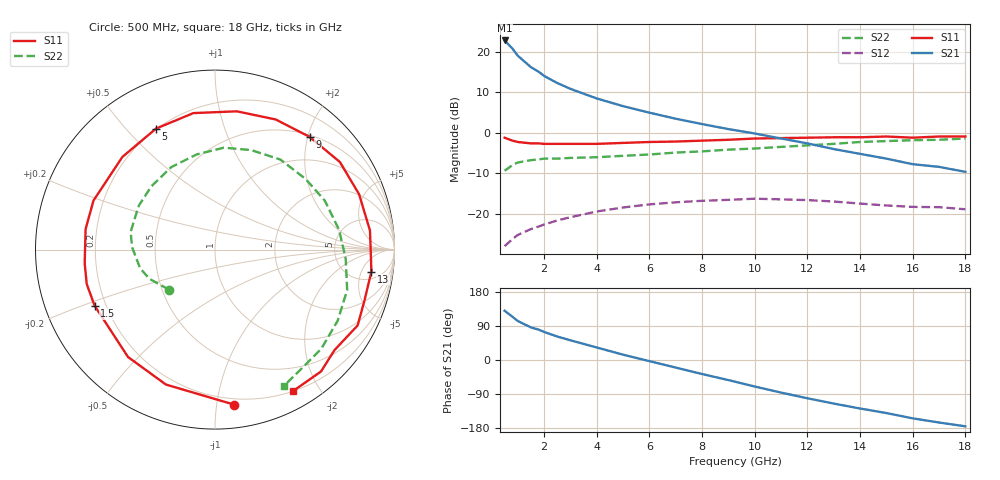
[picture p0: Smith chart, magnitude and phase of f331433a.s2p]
!ATF-33143
!S-PARAMETERS at Vds=3V  Id=60mA.  LAST UPDATED 09-29-99
# ghz s ma r 50
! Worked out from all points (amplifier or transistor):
!   23 points, 500 MHz to 18 GHz, reference 50 ohm
!   highest |S21| = 22.8 dB at 500 MHz (marker M1)
!   |S21| within 3 dB of that: start of sweep to 912.4 MHz
!   unconditionally stable (mu >= 1): 3.853 GHz to end of sweep
!   at 1.5 GHz: K = 0.66, MSG = 20.0 dB, |S12| = -23.7 dB
!   at 7 GHz: K = 1.12, MAG = 8.2 dB, |S12| = -17.1 dB
!   at 18 GHz: K = 1.44, MAG = 0.7 dB, |S12| = -18.9 dB
!   lowest NFmin = 0.11 dB at 500 MHz
!   S11 on the Smith chart (normalised r, x): 500 MHz: 0.16, -1.12; 1.5 GHz: 0.16, -0.22; 5 GHz: 0.20, +0.61; 9 GHz: 0.53, +2.03; 13 GHz: 7, -8; 18 GHz: 0.20, -1.68
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0.5  0.87 -83.0  13.75 130.0  0.04 52.0  0.34 -139.0
0.8  0.8 -110.0  10.89 114.0  0.049 43.0  0.4 -156.0
1  0.77 -129.0  8.92 103.0  0.055 38.0  0.43 -166.0
1.5  0.74 -155.0  6.44 86.0  0.065 32.0  0.46 179.0
1.8  0.74 -165.0  5.64 80.0  0.07 30.0  0.47 173.0
2  0.73 -174.0  5.02 74.0  0.074 29.0  0.48 168.0
2.5  0.73 171.0  4.11 62.0  0.083 25.0  0.48 158.0
3  0.73 158.0  3.48 52.0  0.091 20.0  0.49 150.0
4  0.73 135.0  2.65 33.0  0.107 11.0  0.5 135.0
5  0.75 116.0  2.13 14.0  0.12 0.0  0.52 118.0
6  0.77 99.0  1.77 -3.0  0.131 -12.0  0.54 101.0
7  0.78 81.0  1.49 -20.0  0.139 -25.0  0.57 85.0
8  0.8 65.0  1.28 -37.0  0.145 -37.0  0.59 70.0
9  0.82 50.0  1.11 -53.0  0.149 -50.0  0.62 54.0
10  0.85 35.0  0.98 -70.0  0.154 -63.0  0.64 38.0
11  0.86 21.0  0.85 -86.0  0.151 -76.0  0.67 24.0
12  0.87 7.0  0.74 -101.0  0.148 -88.0  0.7 9.0
13  0.88 -8.0  0.63 -115.0  0.142 -100.0  0.73 -4.0
15  0.9 -28.0  0.48 -140.0  0.127 -120.0  0.79 -30.0
16  0.87 -40.0  0.41 -154.0  0.122 -131.0  0.81 -43.0
17  0.9 -49.0  0.38 -165.0  0.121 -141.0  0.82 -54.0
18  0.9 -61.0  0.33 -175.0  0.114 -149.0  0.85 -63.0
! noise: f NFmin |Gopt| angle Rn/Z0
0.5  0.11  0.72  38  0.07
0.9  0.15  0.66  58  0.07
1.5  0.22  0.57  86  0.05
1.8  0.26  0.52  101  0.05
2.5  0.35  0.43  133  0.03
3  0.42  0.4  154  0.03
5  0.7  0.42  -140  0.06
6  0.84  0.49  -114  0.12
8  1.12  0.64  -74  0.38
10  1.4  0.65  -41  0.82
